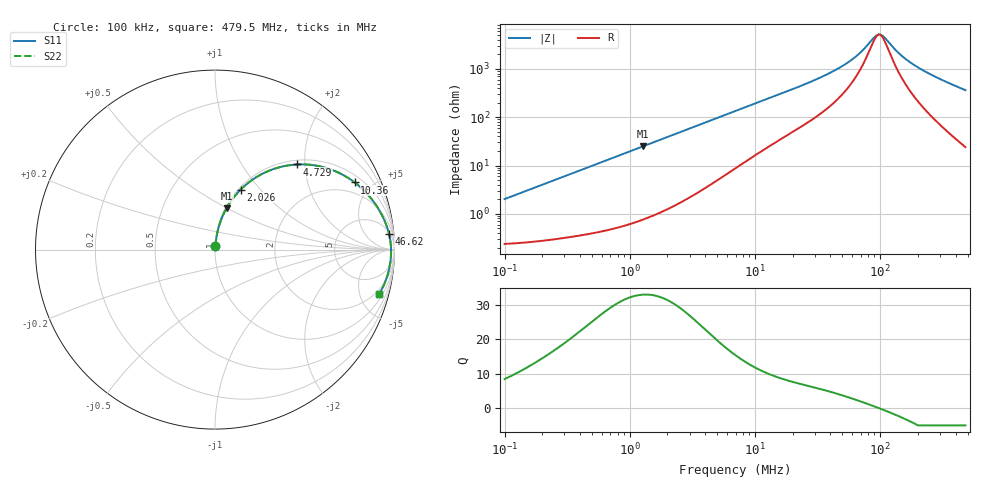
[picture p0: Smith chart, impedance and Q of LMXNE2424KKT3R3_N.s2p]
! LMXNE2424KKT3R3_N  S-PARAMETER MODEL  ( General Type )
! Model Generated by TAIYO YUDEN Corporation (https://www.yuden.co.jp/en/)
! Version 1.0
! TAIYO YUDEN Control No. 191023NI43SB-FBB
! Copyright(c) 2019 TAIYO YUDEN CO.,LTD. All Rights Reserved.
! Product Description (link to TY-COMPAS)
! https://ds.yuden.co.jp/TYCOMPAS/or/detail?pn=LMXNE2424KKT3R3MN&u=M
! Products Name : Inductors
! Characteristics :
!  Inductance : 3.3 uH , SRF(min) : 56 MHz , DC Resistance(max) : 0.264 Ohm
!  Rated Current : Saturation :1000 mA , Temp Rise : 770 mA (40 degC)
!  Case Size : 2.4 x 2.4 / 0.095 x 0.095 [mm/inch] , Thickness : 1 / 0.039 [mm/inch]
!  (Conditions: Temperature = 25 degC , DC Bias Current/Voltage = 0A / 0V)
! External Node Assignments :
!  1  o---GGG---o  2
! GND o---------o GND
! Frequency Range : 0.1MHz  -  479.524407MHz  [ 402 STEP ]
# MHz S RI R 50
! Freq[MHz].  S11 Real  S11 Imag  S21 Real  S21 Imag  S12 Real  S12 Imag  S22 Real  S22 Imag
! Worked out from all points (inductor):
!   401 points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, 100 kHz to 479.5 MHz, reference 50 ohm
!   read as one part in series: L = 3.19 uH near 104.3 kHz
!   highest Q = 32.9 at 1.271 MHz (marker M1), where L = 3.12 uH
!   self-resonance near 98.07 MHz
!   S11 on the Smith chart (normalised r, x): 100 kHz: 1.00, +0.04; 2.026 MHz: 1.03, +0.79; 4.729 MHz: 1.09, +1.83; 10.36 MHz: 1.34, +3.96; 46.62 MHz: 6, +20; 479.5 MHz: 1.48, -7.26
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0.1  0.00277 0.0199  0.9972 -0.0199  0.9972 -0.0199  0.00277 0.0199
0.413557  0.0102 0.0807  0.9898 -0.0807  0.9898 -0.0807  0.0102 0.0807
0.748501  0.0258 0.1427  0.9742 -0.1427  0.9742 -0.1427  0.0258 0.1427
1.271286  0.0646 0.231  0.9354 -0.231  0.9354 -0.231  0.0646 0.231
1.710297  0.1078 0.295  0.8922 -0.295  0.8922 -0.295  0.1078 0.295
2.026226  0.1431 0.3345  0.8569 -0.3345  0.8569 -0.3345  0.1431 0.3345
3.030584  0.2658 0.4235  0.7342 -0.4235  0.7342 -0.4235  0.2658 0.4235
4.728995  0.459 0.4744  0.541 -0.4744  0.541 -0.4744  0.459 0.4744
7.073061  0.6421 0.4477  0.3579 -0.4477  0.3579 -0.4477  0.6421 0.4477
10.35724  0.7785 0.3741  0.2215 -0.3741  0.2215 -0.3741  0.7785 0.3741
16.50777  0.8824 0.2687  0.1176 -0.2687  0.1176 -0.2687  0.8824 0.2687
28.6379  0.9443 0.1621  0.0557 -0.1621  0.0557 -0.1621  0.9443 0.1621
46.62166  0.9693 0.0887  0.0307 -0.0887  0.0307 -0.0887  0.9693 0.0887
65.43652  0.9775 0.0461  0.0225 -0.0461  0.0225 -0.0461  0.9775 0.0461
93.81119  0.9809 0.00497  0.0191 -0.00497  0.0191 -0.00497  0.9809 0.00497
97.87206  0.9811 0.000222  0.0189 -0.000222  0.0189 -0.000222  0.9811 0.000222
104.2953  0.9812 -0.00692  0.0188 0.00692  0.0188 0.00692  0.9812 -0.00692
118.4342  0.981 -0.0213  0.019 0.0213  0.019 0.0213  0.981 -0.0213
149.52  0.9794 -0.0488  0.0206 0.0488  0.0206 0.0488  0.9794 -0.0488
196.9362  0.9747 -0.0845  0.0253 0.0845  0.0253 0.0845  0.9747 -0.0845
294.5534  0.9596 -0.1472  0.0404 0.1472  0.0404 0.1472  0.9596 -0.1472
479.5244  0.9157 -0.2466  0.0843 0.2466  0.0843 0.2466  0.9157 -0.2466
